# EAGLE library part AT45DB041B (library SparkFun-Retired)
4-Mbit SPI flash memory Not in catalog
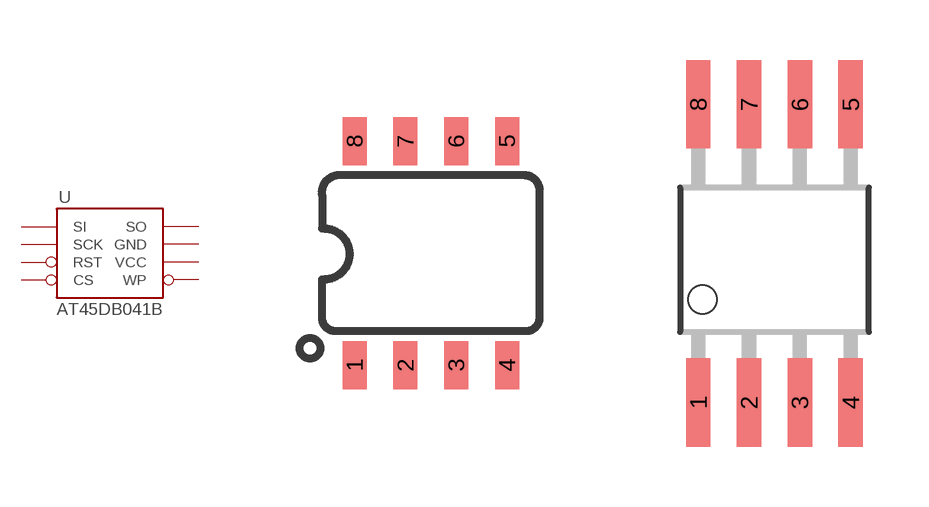
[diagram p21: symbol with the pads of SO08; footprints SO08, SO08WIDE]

Designator prefix -

## AT45DB041B  [SO08]
1  SI
2  SCK
3  RST
4  CS
5  WP
6  VCC
7  GND
8  SO

## AT45DB041BWIDE  [SO08WIDE]
Pads as for SO08

## Footprint SO08 (pad centres in mm)
SOIC, 0.15 inch width
smd 0.6 x 1.2: 1 -1.905,-2.8; 2 -0.635,-2.8; 3 0.635,-2.8; 4 1.905,-2.8; 5 1.905,2.8; 6 0.635,2.8; 7 -0.635,2.8; 8 -1.905,2.8

## Footprint SO08WIDE (pad centres in mm)
smd 0.61 x 2.21: 1 -1.905,-3.569; 2 -0.635,-3.569; 3 0.635,-3.569; 4 1.905,-3.569; 5 1.905,3.886; 6 0.635,3.886; 7 -0.635,3.886; 8 -1.905,3.886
